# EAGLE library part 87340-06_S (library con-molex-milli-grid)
RECEPTACAL
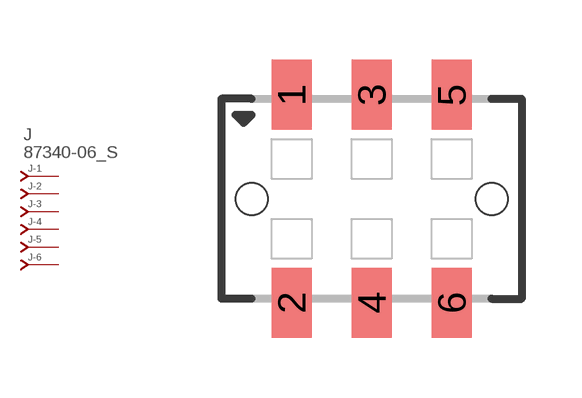
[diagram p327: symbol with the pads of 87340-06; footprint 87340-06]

Designator prefix J; gates -1=J-NV -2=J-N -3=J-N -4=J-N -5=J-N -6=J-N

## 87340-06_S  [87340-06]
1  -1:J  pas
2  -2:J  pas
3  -3:J  pas
4  -4:J  pas
5  -5:J  pas
6  -6:J  pas

## Footprint 87340-06 (pad centres in mm)
RECEPTACAL SMD Dual Row, Vertical, Low Profile
smd 1 x 1.75: 1 -2,2.6; 2 -2,-2.6; 3 0,2.6; 4 0,-2.6; 5 2,2.6; 6 2,-2.6
hole 0.8 at -3,0
hole 0.8 at 3,0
